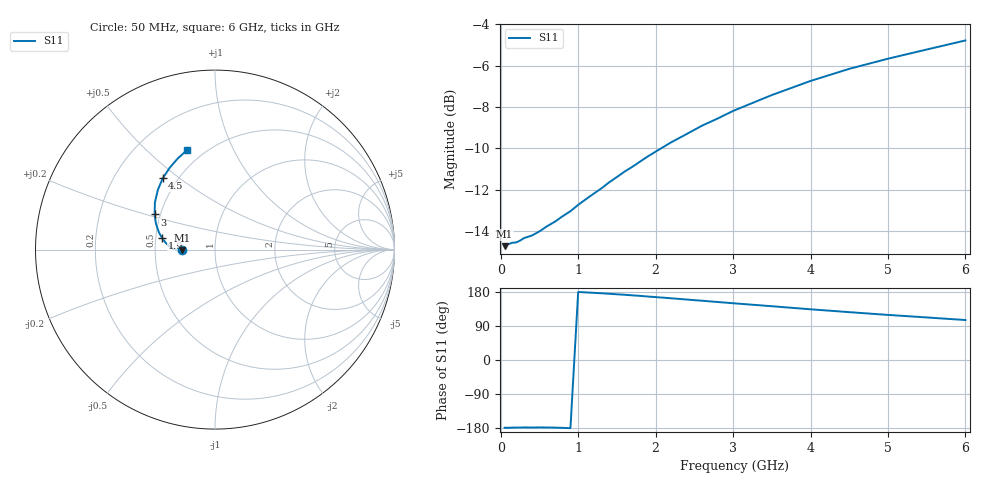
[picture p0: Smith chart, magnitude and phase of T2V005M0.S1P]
! SIEMENS Discrete & RF Semiconductors
! BAS70-04W
! Si Schottky Diode in SOT323
! IF = 5 mA
! S-Parameters:  November  1997
# GHz  S  MA  R  50
!  f  S11
! GHz  MAG  ANG
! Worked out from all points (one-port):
!   34 points, 50 MHz to 6 GHz, reference 50 ohm
!   lowest |S11| = -14.7 dB at 50 MHz (marker M1), VSWR 1.45, Z = 34.5 - j0.251 ohm
!   |S11| at or under -10 dB: start of sweep to 2.073 GHz
!   S11 on the Smith chart (normalised r, x): 50 MHz: 0.69, -0.01; 1.9 GHz: 0.54, +0.08; 3 GHz: 0.46, +0.21; 4.5 GHz: 0.42, +0.43; 6 GHz: 0.41, +0.68
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0.05  0.1832 -178.9
0.15  0.1867 -178.4
0.2  0.1871 -178.2
0.3  0.1916 -177.9
0.4  0.1943 -178.1
0.5  0.1989 -177.9
0.6  0.2049 -178.1
0.7  0.21 -178.4
0.8  0.2165 -179.1
0.9  0.2226 -179.9
1  0.2307 179.4
1.1  0.2381 178.4
1.3  0.2529 176.1
1.4  0.2615 174.8
1.6  0.2777 172.1
1.8  0.2937 169.2
1.9  0.3023 167.5
2.2  0.3268 162.9
2.4  0.3423 159.6
2.6  0.3588 156.4
2.8  0.3732 153.1
3  0.3893 149.8
3.5  0.4254 141.9
4  0.4602 133.8
4.5  0.4924 126.3
5  0.521 119.0
5.5  0.5483 112.3
6  0.5768 105.5
